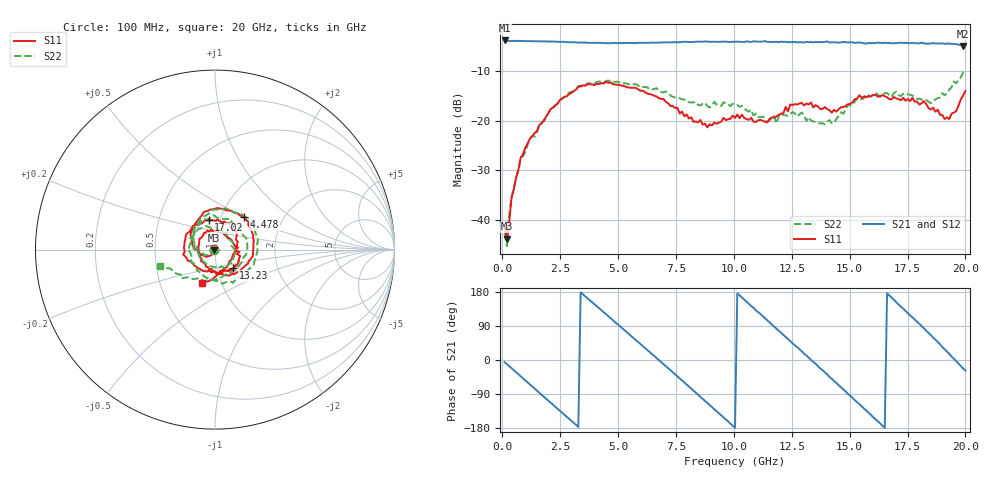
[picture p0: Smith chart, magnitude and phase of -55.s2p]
!Agilent Technologies,N5230C,MY49001569,A.09.33.09
!Agilent N5230C: A.09.33.09
!Date: Wednesday, July 29, 2015 16:27:02
!Correction: S11(Full 2 Port(1,2))
!S21(Full 2 Port(1,2))
!S12(Full 2 Port(1,2))
!S22(Full 2 Port(1,2))
!S2P File: Measurements: S11, S21, S12, S22:
# Hz S  dB  R 50
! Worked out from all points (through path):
!   201 points, 100 MHz to 20 GHz, reference 50 ohm
!   highest |S21| = -3.92 dB at 100 MHz (marker M1); lowest = -5.0 dB at 19.9 GHz (marker M2)
!   group delay of S21, straight-line fit = 152 ps
!   lowest |S11| = -43.7 dB at 199.5 MHz (marker M3), VSWR 1.01, Z = 49.5 - j0.464 ohm
!   |S11| at or under -10 dB: start of sweep to end of sweep
!   |S22| runs from -45.2 to -9.8 dB; largest |S21 - S12| = 0.024
!   S11 on the Smith chart (normalised r, x): 100 MHz: 0.98, +0.00; 4.478 GHz: 1.28, +0.50; 13.23 GHz: 1.20, -0.25; 17.02 GHz: 0.89, +0.30; 20 GHz: 0.81, -0.31
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1e8  -41.56 174.0  -3.92 -5.7  -3.92 -5.8  -42.71 -161.7
1.995e8  -43.73 -134.0  -3.99 -10.9  -4.03 -11.0  -45.22 -100.5
3.985e8  -35.50 -105.7  -4.04 -21.6  -4.03 -21.8  -35.41 -109.1
7.965e8  -27.37 -127.3  -4.04 -43.0  -4.04 -43.1  -27.63 -129.8
1.7915e9  -19.96 -178.2  -4.12 -96.9  -4.12 -96.9  -20.15 177.9
3.483e9  -12.94 96.0  -4.36 173.3  -4.35 173.1  -13.03 87.1
4.478e9  -12.23 48.1  -4.49 120.8  -4.46 120.6  -12.07 36.6
5.473e9  -13.39 2.4  -4.42 68.5  -4.46 68.1  -12.72 -8.5
6.7665e9  -15.52 -53.1  -4.35 -0.4  -4.37 -0.9  -14.04 -63.8
8.458e9  -20.37 -132.0  -4.16 -91.6  -4.18 -92.2  -16.90 -135.7
1.005e10  -19.49 119.2  -4.19 -179.0  -4.22 -179.0  -16.70 128.0
1.1642e10  -19.37 29.4  -4.22 93.5  -4.18 93.7  -19.41 21.9
1.3234e10  -16.78 -44.8  -4.27 5.8  -4.28 5.4  -19.33 -80.3
1.3433e10  -17.37 -56.4  -4.30 -5.1  -4.31 -5.6  -20.19 -92.2
1.5025e10  -16.67 -148.6  -4.30 -94.4  -4.31 -95.1  -16.96 156.0
1.5821e10  -15.16 166.7  -4.39 -139.1  -4.42 -140.4  -14.96 109.8
1.67165e10  -15.74 117.5  -4.41 170.4  -4.49 169.4  -14.93 59.6
1.7015e10  -15.55 102.1  -4.47 152.3  -4.49 152.5  -14.25 41.3
1.8408e10  -17.51 28.2  -4.55 71.5  -4.43 70.1  -16.23 -55.7
1.93035e10  -19.71 -38.2  -4.54 16.4  -4.68 14.8  -13.81 -126.1
1.99005e10  -14.99 -100.6  -5.03 -22.4  -4.94 -23.6  -10.39 -159.7
2e10  -14.06 -111.5  -4.89 -27.7  -5.03 -29.0  -9.82 -163.2
